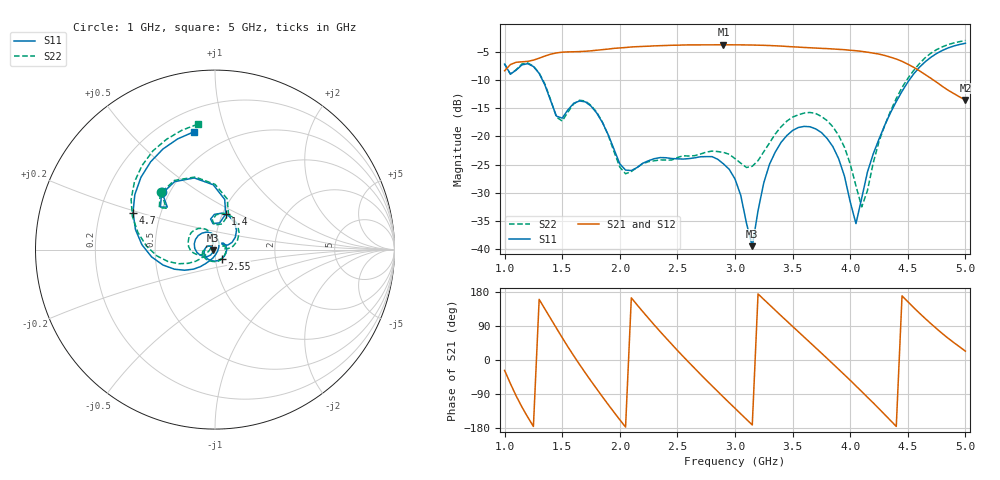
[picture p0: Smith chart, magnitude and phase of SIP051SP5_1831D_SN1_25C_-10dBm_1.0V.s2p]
# GHz  S  dB  R  50
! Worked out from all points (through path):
!   81 points, 1 GHz to 5 GHz, reference 50 ohm
!   highest |S21| = -3.78 dB at 2.9 GHz (marker M1); lowest = -13.5 dB at 5 GHz (marker M2)
!   lowest |S11| = -39.4 dB at 3.15 GHz (marker M3), VSWR 1.02, Z = 49 - j0.278 ohm
!   |S11| at or under -10 dB: 1.328 GHz to 4.514 GHz (3.186 GHz wide, 109 % of centre)
!   |S22| runs from -32.5 to -3.0 dB; largest |S21 - S12| = 0.0044
!   S11 on the Smith chart (normalised r, x): 1 GHz: 0.45, +0.36; 1.4 GHz: 1.04, +0.43; 2.55 GHz: 1.07, -0.11; 4.7 GHz: 0.35, +0.19; 5 GHz: 0.33, +0.78
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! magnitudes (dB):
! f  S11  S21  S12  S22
! 1 GHz  -7.2  -8.4  -8.4  -7.2
! 1.25 GHz  -7.6  -6.5  -6.5  -7.5
! 1.4 GHz  -13.7  -5.4  -5.4  -13.5
! 1.5 GHz  -16.8  -5.1  -5.1  -17.3
! 1.7 GHz  -13.9  -4.9  -4.9  -13.7
! 2.05 GHz  -26.0  -4.3  -4.3  -26.6
! 2.35 GHz  -23.7  -3.9  -3.9  -24.2
! 2.55 GHz  -24.0  -3.8  -3.8  -23.4
! 2.9 GHz  -24.9  -3.8  -3.8  -22.8
! 3 GHz  -27.5  -3.8  -3.8  -23.9
! 3.15 GHz  -39.4  -3.8  -3.8  -25.3
! 3.25 GHz  -28.2  -3.9  -3.9  -22.7
! 3.35 GHz  -22.7  -4.0  -4.0  -19.5
! 3.5 GHz  -18.9  -4.1  -4.1  -16.6
! 3.7 GHz  -18.7  -4.4  -4.4  -15.9
! 3.9 GHz  -24.0  -4.6  -4.6  -19.8
! 4.05 GHz  -35.4  -4.8  -4.8  -28.7
! 4.1 GHz  -30.9  -5.0  -4.9  -32.5
! 4.2 GHz  -23.1  -5.3  -5.3  -24.7
! 4.35 GHz  -15.8  -6.0  -6.0  -15.5
! 4.7 GHz  -6.0  -9.7  -9.7  -5.3
! 5 GHz  -3.5  -13.5  -13.5  -3.0
